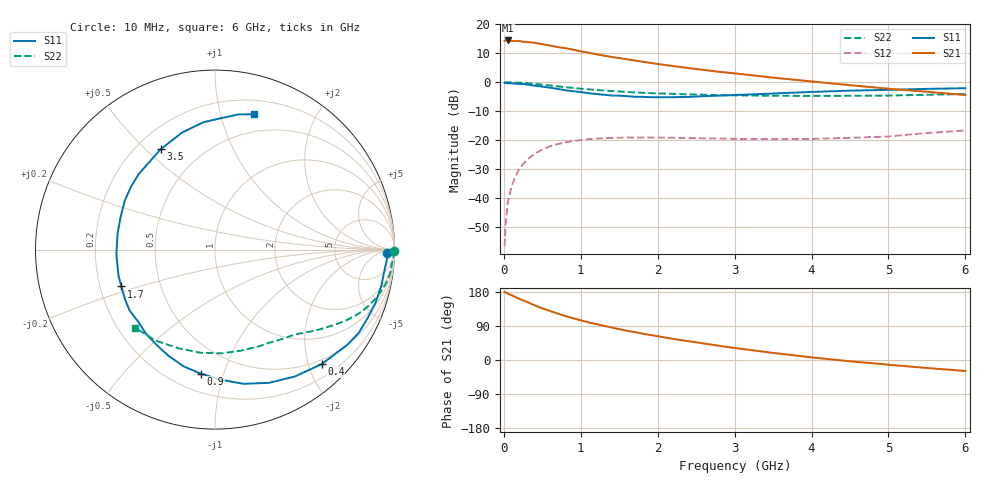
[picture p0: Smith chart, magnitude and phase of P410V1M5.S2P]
! SIEMENS Small Signal Semiconductors
! BFP182
! Si NPN RF Bipolar Junction Transistor in SOT143
! VCE = 10 V  IC = 1.5 mA
! Common Emitter S-Parameters:  March  1996
# GHz  S  MA  R  50
!  f  S11  S21  S12  S22
! GHz  MAG  ANG  MAG  ANG  MAG  ANG  MAG  ANG
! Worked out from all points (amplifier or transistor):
!   36 points, 10 MHz to 6 GHz, reference 50 ohm
!   highest |S21| = 14.3 dB at 50 MHz (marker M1)
!   |S21| within 3 dB of that: start of sweep to 866.7 MHz
!   unconditionally stable (mu >= 1): 2.441 GHz to end of sweep
!   at 250 MHz: K = 0.12, MSG = 21.1 dB, |S12| = -28.2 dB
!   at 1.4 GHz: K = 0.60, MSG = 13.9 dB, |S12| = -19.2 dB
!   at 6 GHz: K = 1.05, MAG = 4.8 dB, |S12| = -16.7 dB
!   S11 on the Smith chart (normalised r, x): 10 MHz: 40, -19; 400 MHz: 0.42, -2.23; 900 MHz: 0.31, -0.84; 1.7 GHz: 0.29, -0.17; 3.5 GHz: 0.30, +0.56; 6 GHz: 0.33, +1.28
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0.01  0.9601 -1.1  5.123 179.2  0.0015 84.3  0.996 -0.4
0.02  0.9616 -2.7  5.191 178.6  0.0032 88.5  0.9959 -1.0
0.05  0.9524 -6.2  5.209 175.4  0.0083 86.9  0.995 -2.3
0.1  0.9485 -12.0  5.095 171.0  0.0159 81.8  0.9878 -4.6
0.15  0.9426 -18.3  5.121 166.3  0.0238 77.7  0.9864 -7.0
0.2  0.9318 -24.3  5.102 161.6  0.0318 75.8  0.9787 -9.3
0.4  0.8719 -47.1  4.757 144.2  0.0582 61.9  0.9324 -17.5
0.5  0.8351 -57.9  4.483 136.3  0.0689 55.7  0.9027 -21.1
0.6  0.8005 -68.0  4.259 129.3  0.0787 50.4  0.8753 -24.1
0.8  0.7253 -87.6  3.829 116.0  0.0918 40.9  0.8192 -29.4
0.9  0.6961 -96.4  3.619 110.2  0.0971 37.0  0.7924 -31.6
1.1  0.6455 -113.8  3.206 99.3  0.1043 30.2  0.7503 -35.5
1.4  0.5874 -136.5  2.707 85.8  0.1095 22.2  0.7038 -40.3
1.7  0.5604 -158.5  2.356 73.6  0.1108 16.9  0.6641 -44.7
1.9  0.5505 -171.2  2.143 66.2  0.1111 14.0  0.647 -47.6
2.2  0.5498 171.3  1.889 55.7  0.1101 10.9  0.6276 -51.9
2.8  0.585 143.0  1.503 37.4  0.107 7.8  0.5969 -61.5
3.5  0.6358 118.4  1.193 18.7  0.104 8.0  0.5817 -75.0
4  0.6772 105.8  1.027 7.0  0.1054 10.2  0.5792 -86.0
4.5  0.7126 95.2  0.884 -3.4  0.1098 12.0  0.5807 -98.0
5.5  0.7649 80.1  0.682 -21.1  0.133 16.2  0.6056 -123.2
6  0.7849 73.8  0.599 -29.0  0.1468 14.2  0.623 -135.7
